FUNCTION "IndicationLoader" : VOID
TITLE =
VERSION : 0.1

BEGIN
NETWORK
TITLE =Indication start auto loaderside
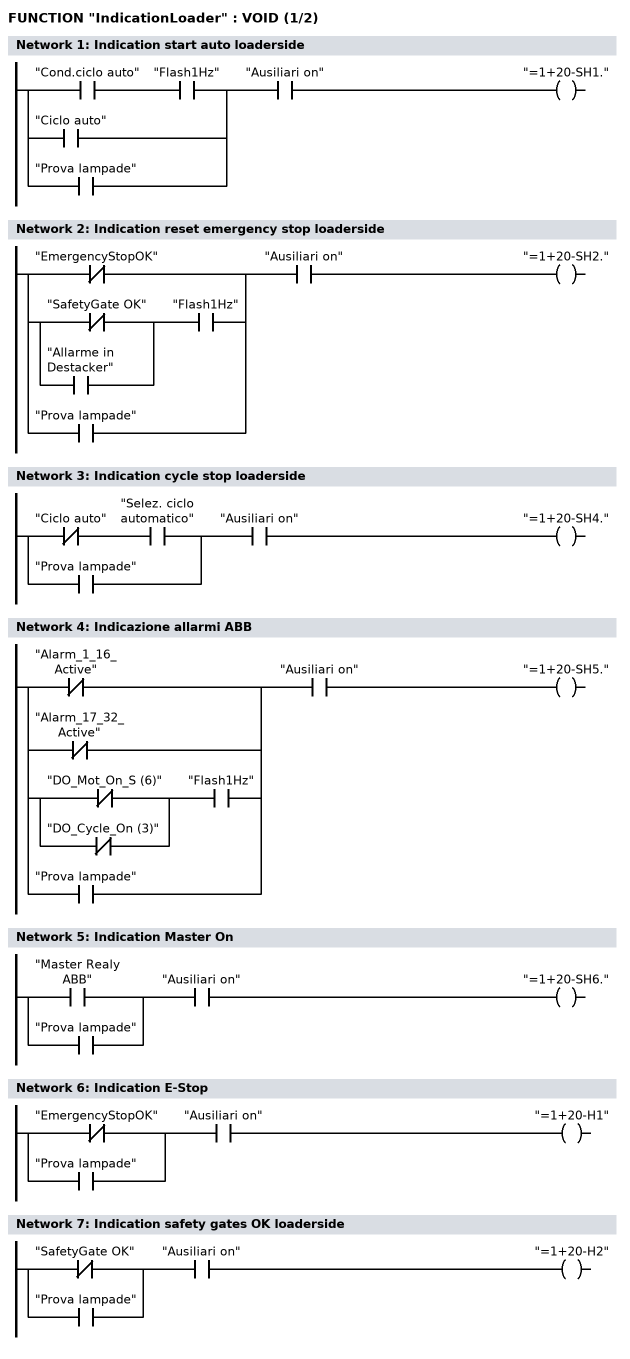
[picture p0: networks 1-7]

      U(    ;
      U     "Cond.ciclo auto";
      U     "Flash1Hz";
      O     "Ciclo auto";
      O     "Prova lampade";
      )     ;
      U     "Ausiliari on";
      =     "=1+20-SH1.";
NETWORK
TITLE =Indication reset emergency stop loaderside

      U(    ;
      ON    "EmergencyStopOK";
      O     ;
      U(    ;
      ON    "SafetyGate OK";
      O     "Allarme in Destacker";
      )     ;
      U     "Flash1Hz";
      O     "Prova lampade";
      )     ;
      U     "Ausiliari on";
      =     "=1+20-SH2.";
NETWORK
TITLE =Indication cycle stop loaderside

      U(    ;
      UN    "Ciclo auto";
      U     "Selez. ciclo automatico";
      O     "Prova lampade";
      )     ;
      U     "Ausiliari on";
      =     "=1+20-SH4.";
NETWORK
TITLE =Indicazione allarmi ABB

      U(    ;
      ON    "Alarm_1_16_Active";
      ON    "Alarm_17_32_Active";
      O     ;
      U(    ;
      ON    "DO_Mot_On_S (6)";
      ON    "DO_Cycle_On (3)";
      )     ;
      U     "Flash1Hz";
      O     "Prova lampade";
      )     ;
      U     "Ausiliari on";
      =     "=1+20-SH5.";
NETWORK
TITLE =Indication Master On

      U(    ;
      O     "Master Realy ABB";
      O     "Prova lampade";
      )     ;
      U     "Ausiliari on";
      =     "=1+20-SH6.";
NETWORK
TITLE =Indication E-Stop

      U(    ;
      ON    "EmergencyStopOK";
      O     "Prova lampade";
      )     ;
      U     "Ausiliari on";
      =     "=1+20-H1";
NETWORK
TITLE =Indication safety gates OK loaderside

      U(    ;
      ON    "SafetyGate OK";
      O     "Prova lampade";
      )     ;
      U     "Ausiliari on";
      =     "=1+20-H2";
NETWORK
TITLE =Indication arm safety loader
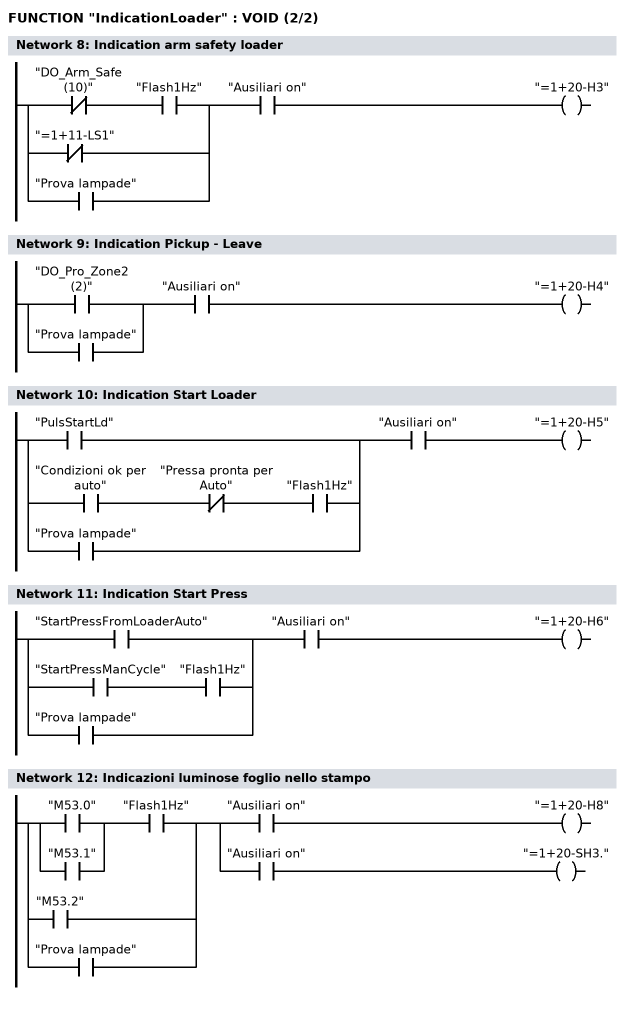
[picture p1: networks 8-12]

      U(    ;
      UN    "DO_Arm_Safe (10)";
      U     "Flash1Hz";
      ON    "=1+11-LS1";
      O     "Prova lampade";
      )     ;
      U     "Ausiliari on";
      =     "=1+20-H3";
NETWORK
TITLE =Indication Pickup - Leave

      U(    ;
      O     "DO_Pro_Zone2 (2)";
      O     "Prova lampade";
      )     ;
      U     "Ausiliari on";
      =     "=1+20-H4";
NETWORK
TITLE =Indication Start Loader

      U(    ;
      O     "PulsStartLd";
      O     ;
      U     "Condizioni ok per auto";
      UN    "Pressa pronta per Auto";
      U     "Flash1Hz";
      O     "Prova lampade";
      )     ;
      U     "Ausiliari on";
      =     "=1+20-H5";
NETWORK
TITLE =Indication Start Press

      U(    ;
      O     "StartPressFromLoaderAuto";
      O     ;
      U     "StartPressManCycle";
      U     "Flash1Hz";
      O     "Prova lampade";
      )     ;
      U     "Ausiliari on";
      =     "=1+20-H6";
NETWORK
TITLE =Indicazioni luminose foglio nello stampo

      U(    ;
      O     "M53.0";
      O     "M53.1";
      )     ;
      U     "Flash1Hz";
      O     "M53.2";
      O     "Prova lampade";
      =     L      0.0;
      U     L      0.0;
      U     "Ausiliari on";
      =     "=1+20-H8";
      U     L      0.0;
      U     "Ausiliari on";
      =     "=1+20-SH3.";
END_FUNCTION

